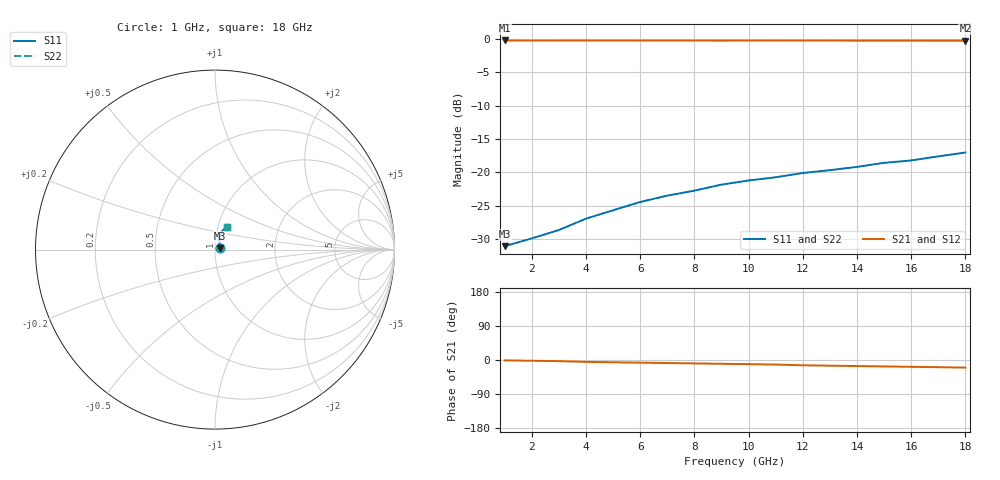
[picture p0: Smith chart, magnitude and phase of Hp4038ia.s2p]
!HPND-4038 beam lead PIN diode
!Series configuration S-parameters If= 1 mA.  Last updated 10/3/97
# mhz s ma r 50
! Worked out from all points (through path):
!   18 points, 1 GHz to 18 GHz, reference 50 ohm
!   highest |S21| = -0.21 dB at 1 GHz (marker M1); lowest = -0.2 dB at 18 GHz (marker M2)
!   group delay of S21, straight-line fit = 3.13 ps
!   lowest |S11| = -31.1 dB at 1 GHz (marker M3), VSWR 1.06, Z = 52.8 + j0.766 ohm
!   |S11| at or under -10 dB: start of sweep to end of sweep
!   |S22| runs from -31.1 to -17.0 dB; largest |S21 - S12| = 0
1000  0.028 15.0  0.976 -1.0  0.976 -1.0  0.028 15.0
2000  0.032 34.0  0.974 -2.0  0.974 -2.0  0.032 34.0
3000  0.037 47.0  0.975 -3.0  0.975 -3.0  0.037 47.0
4000  0.045 55.0  0.975 -5.0  0.975 -5.0  0.045 55.0
5000  0.052 61.0  0.974 -6.0  0.974 -6.0  0.052 61.0
6000  0.06 65.0  0.974 -7.0  0.974 -7.0  0.06 65.0
7000  0.067 67.0  0.974 -8.0  0.974 -8.0  0.067 67.0
8000  0.073 69.0  0.974 -9.0  0.974 -9.0  0.073 69.0
9000  0.081 70.0  0.973 -10.0  0.973 -10.0  0.081 70.0
10000  0.087 71.0  0.974 -11.0  0.974 -11.0  0.087 71.0
11000  0.092 71.0  0.975 -12.0  0.975 -12.0  0.092 71.0
12000  0.099 70.0  0.974 -14.0  0.974 -14.0  0.099 70.0
13000  0.104 70.0  0.975 -15.0  0.975 -15.0  0.104 70.0
14000  0.11 69.0  0.972 -16.0  0.972 -16.0  0.11 69.0
15000  0.118 67.0  0.973 -17.0  0.973 -17.0  0.118 67.0
16000  0.123 66.0  0.973 -18.0  0.973 -18.0  0.123 66.0
17000  0.132 64.0  0.972 -19.0  0.972 -19.0  0.132 64.0
18000  0.141 62.0  0.972 -20.0  0.972 -20.0  0.141 62.0
